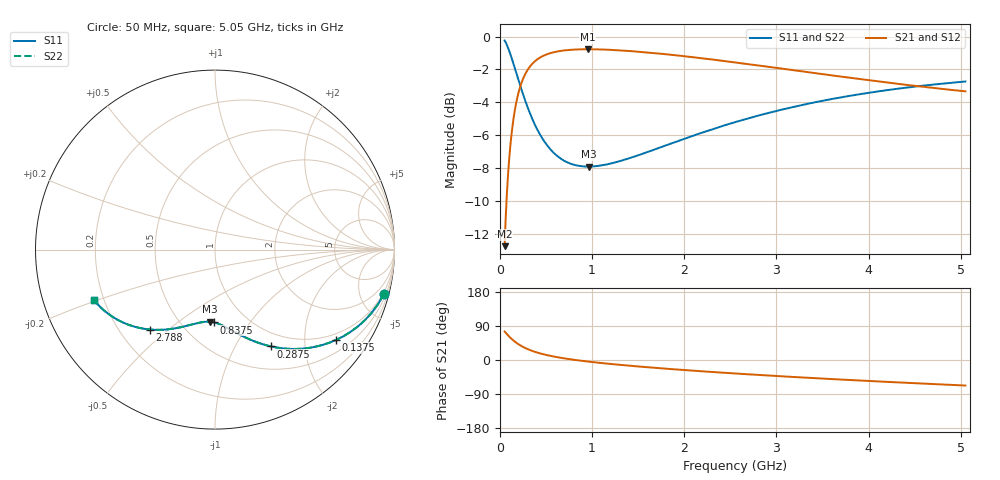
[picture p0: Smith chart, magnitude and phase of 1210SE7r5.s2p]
! AVX Thin Film Operation		Date: August 2001
! Description: Accu-P® Series, Thin Film, SMD, RF Capacitor
! Part Number: 12101J7R5BBT
! 50 MHz  -  5.05 GHz
! Serial Measurements
# mhz S db R 50
!	S11		S21		S12		S22
!	dB	Phase	dB	Phase	dB	Phase	dB	Phase
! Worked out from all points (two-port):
!   401 points, 50 MHz to 5.05 GHz, reference 50 ohm
!   highest |S21| = -0.77 dB at 950 MHz (marker M1); lowest = -12.7 dB at 50 MHz (marker M2)
!   |S21| within 3 dB of the highest: 185.4 MHz to end of sweep
!   lowest |S11| = -7.9 dB at 962.5 MHz (marker M3), VSWR 2.35, Z = 34.2 - j32.9 ohm
!   |S11| at or under -10 dB: nowhere
!   |S22| runs from -7.9 to -0.2 dB; largest |S21 - S12| = 0
!   S11 on the Smith chart (normalised r, x): 50 MHz: 0.81, -7.59; 137.5 MHz: 0.81, -2.80; 287.5 MHz: 0.80, -1.41; 837.5 MHz: 0.71, -0.69; 2.788 GHz: 0.33, -0.43; 5.05 GHz: 0.16, -0.20
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50  -0.24 -14.8  -12.72 75.2  -12.72 75.2  -0.24 -14.8
75  -0.52 -21.8  -9.51 68.2  -9.51 68.2  -0.52 -21.8
100  -0.87 -28.2  -7.41 61.8  -7.41 61.8  -0.87 -28.2
137.5  -1.50 -36.7  -5.35 53.2  -5.35 53.2  -1.50 -36.7
200  -2.63 -48.3  -3.43 41.7  -3.43 41.7  -2.63 -48.3
237.5  -3.29 -53.8  -2.75 36.2  -2.75 36.2  -3.29 -53.8
287.5  -4.11 -59.9  -2.14 30.0  -2.14 30.0  -4.11 -59.9
387.5  -5.45 -69.2  -1.46 20.8  -1.46 20.8  -5.45 -69.2
500  -6.52 -76.6  -1.10 13.4  -1.10 13.4  -6.52 -76.6
650  -7.38 -83.8  -0.88 6.2  -0.88 6.2  -7.38 -83.8
837.5  -7.83 -90.5  -0.78 -0.6  -0.78 -0.6  -7.83 -90.5
887.5  -7.87 -92.1  -0.78 -2.1  -0.78 -2.1  -7.87 -92.1
950  -7.89 -93.9  -0.77 -4.0  -0.77 -4.0  -7.89 -93.9
962.5  -7.89 -94.3  -0.77 -4.3  -0.77 -4.3  -7.89 -94.3
1325  -7.52 -103.3  -0.85 -13.3  -0.85 -13.3  -7.52 -103.3
1725  -6.76 -111.5  -1.03 -21.5  -1.03 -21.5  -6.76 -111.5
2125  -5.96 -118.7  -1.27 -28.7  -1.27 -28.7  -5.96 -118.7
2550  -5.20 -125.6  -1.57 -35.6  -1.57 -35.6  -5.20 -125.6
2787.5  -4.82 -129.1  -1.74 -39.2  -1.74 -39.2  -4.82 -129.1
3387.5  -4.03 -137.5  -2.20 -47.6  -2.20 -47.6  -4.03 -137.5
4225  -3.23 -148.0  -2.81 -58.0  -2.81 -58.0  -3.23 -148.0
5050  -2.73 -157.3  -3.33 -67.3  -3.33 -67.3  -2.73 -157.3
